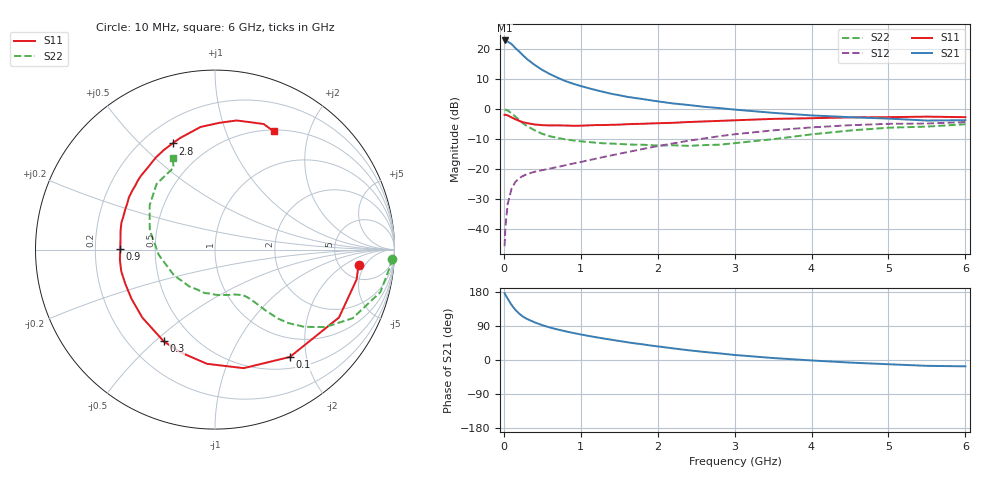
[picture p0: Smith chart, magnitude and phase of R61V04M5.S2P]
! SIEMENS Small Signal Semiconductors
! BFR193
! Si NPN RF Bipolar Junction Transistor in SOT23
! VCE = 1 V  IC = 4.5 mA
! Common Emitter S-Parameters:  May  1996
# GHz  S  MA  R  50
!  f  S11  S21  S12  S22
! GHz  MAG  ANG  MAG  ANG  MAG  ANG  MAG  ANG
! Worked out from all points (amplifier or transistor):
!   36 points, 10 MHz to 6 GHz, reference 50 ohm
!   highest |S21| = 23.0 dB at 10 MHz (marker M1)
!   |S21| within 3 dB of that: start of sweep to 169.3 MHz
!   unconditionally stable (mu >= 1): 891.5 MHz to 2.201 GHz
!   at 250 MHz: K = 0.41, MSG = 20.2 dB, |S12| = -22.3 dB
!   at 1.4 GHz: K = 1.08, MAG = 8.5 dB, |S12| = -15.5 dB
!   at 6 GHz: K = 0.99, MSG = 0.3 dB, |S12| = -4.3 dB
!   S11 on the Smith chart (normalised r, x): 10 MHz: 7.45, -3.61; 100 MHz: 0.67, -1.72; 300 MHz: 0.34, -0.53; 900 MHz: 0.31, +0.00; 2.8 GHz: 0.32, +0.63; 6 GHz: 0.52, +1.49
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0.01  0.8043 -6.1  14.14 176.5  0.0051 86.4  0.9897 -2.9
0.02  0.8064 -11.9  13.89 172.4  0.0106 83.0  0.9784 -5.9
0.05  0.7876 -28.7  13.56 161.7  0.0259 75.2  0.9516 -14.4
0.1  0.7293 -55.1  12.32 145.5  0.0464 64.1  0.8569 -26.5
0.15  0.6796 -76.4  10.55 132.3  0.0608 55.4  0.7521 -35.0
0.2  0.638 -94.0  9.208 122.3  0.0702 49.8  0.6589 -40.8
0.25  0.6037 -108.6  7.954 114.3  0.0764 46.2  0.5793 -45.0
0.3  0.5856 -119.2  6.917 108.5  0.0818 44.1  0.5225 -47.5
0.4  0.5546 -136.8  5.517 99.4  0.0897 42.2  0.4437 -50.2
0.5  0.5402 -149.4  4.536 91.9  0.0954 42.6  0.3873 -52.1
0.6  0.5349 -159.3  3.863 85.7  0.1016 43.7  0.3521 -53.7
0.7  0.5361 -167.1  3.359 80.5  0.1081 45.0  0.33 -55.1
0.9  0.5276 179.8  2.672 71.4  0.123 47.8  0.3007 -58.1
1.1  0.5363 168.8  2.249 63.6  0.1399 50.8  0.2822 -63.1
1.3  0.543 160.0  1.938 56.6  0.1588 52.6  0.2684 -68.3
1.6  0.5608 148.8  1.613 47.0  0.1906 54.0  0.258 -78.2
2.2  0.5918 128.9  1.247 30.7  0.2676 52.0  0.249 -103.4
2.8  0.6372 111.8  1.044 17.5  0.3528 45.2  0.2545 -137.0
3.5  0.6881 96.7  0.869 5.2  0.4425 34.2  0.3148 -174.7
4.5  0.7292 80.6  0.735 -6.8  0.5397 17.5  0.44 145.9
5.5  0.7504 68.8  0.646 -15.4  0.5756 1.4  0.5112 116.8
6  0.7353 63.5  0.655 -16.7  0.6093 -3.3  0.5606 114.9
